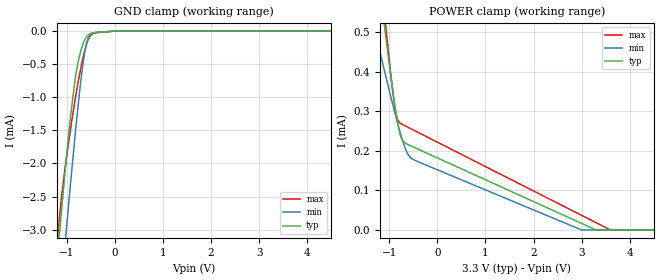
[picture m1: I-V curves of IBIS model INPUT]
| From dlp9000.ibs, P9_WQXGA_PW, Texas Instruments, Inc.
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|   Model
[Model]   INPUT
Model_type   Input
Vinl = 0.7
Vinh = 1.7
|   typ   min   max
C_comp   0.532pF   0.482pF   0.599pF
[Voltage Range]   3.3   3   3.6
[Temperature Range]   25   125   -40
[Power Clamp Reference]   3.3   3   3.6
[GND Clamp Reference]   -0   -0   -0
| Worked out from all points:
|   GND clamp passes 1 mA (typ) near -0.87 V on its own axis
[GND Clamp]
|   Voltage   I(typ)   I(min)   I(max)
-3.3V     -22.6mA    -23.66mA   -24.17mA
-1.221V   -3.646mA   -4.742mA   -3.341mA
-1.122V   -2.815mA   -3.915mA   -2.588mA
-1.023V   -2.02mA    -3.102mA   -1.995mA
-1.003V   -1.867mA   -2.942mA   -1.889mA
-924mV    -1.295mA   -2.311mA   -1.487mA
-795.3mV  -585.5uA   -1.338mA   -897.1uA
-646.8mV  -164.2uA   -408.8uA   -351.4uA
-587.4mV  -83.92uA   -178.8uA   -192.8uA
-518.1mV  -41.13uA   -58.96uA   -78.71uA
-3.3mV    -178.5nA   -163.1nA   -200.2nA
6.59V     0A         0A         0A
[POWER Clamp]
|   Voltage   I(typ)   I(min)   I(max)
-3.3V     2.812mA    1.561mA    3.455mA
-1.419V   836.4uA    564.5uA    954.4uA
-1.28V    695uA      493uA      775.2uA
-1.112V   526.7uA    407.5uA    562.4uA
-1.033V   449.7uA    368uA      466.1uA
-874.5mV  307uA      291.5uA    302.6uA
-765.6mV  237.5uA    242.8uA    269.5uA
-587.4mV  214.6uA    186.8uA    258.1uA
-270.6mV  197.1uA    165.8uA    238.6uA
2.996V    16.75uA    178.1nA    37.18uA
3.59V     0A         0A         588.3nA
6.59V     0A         0A         0A
